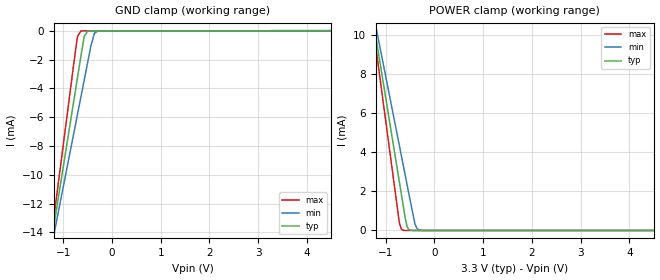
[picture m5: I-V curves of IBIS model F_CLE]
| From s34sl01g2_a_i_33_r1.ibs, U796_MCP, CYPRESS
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|   Model   F_CLE
[Model]   F_CLE
Model_type Input
Vinl =   0.6600V
Vinh =   2.6400V
   C_comp   1.3066pF   1.2854pF   1.3186pF
[Temperature Range]   25.0000   0.1050k   -40.0000
[Pullup Reference]   3.3000V   3.0000V   3.6000V
[Pulldown Reference]   0.0V   0.0V   0.0V
[POWER Clamp Reference]   3.3000V   3.0000V   3.6000V
[GND Clamp Reference]   0.0V   0.0V   0.0V
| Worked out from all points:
|   GND clamp passes 1 mA (typ) near -0.60 V on its own axis
|   POWER clamp passes 1 mA (typ) near -0.62 V on its own axis
[GND_clamp]
|Voltage   I(typ)   I(min)   I(max)
-3.3V     -58.25mA   -50.51mA   -68.01mA
-1.27V    -15.17mA   -15.49mA   -14.97mA
-1.2V     -13.69mA   -14.29mA   -13.14mA
-1.13V    -12.2mA    -13.08mA   -11.31mA
-710mV    -3.287mA   -5.833mA   -406.4uA
-640mV    -1.801mA   -4.625mA   -13.92uA
-570mV    -392.3uA   -3.417mA   -432.3nA
-500mV    -27.95uA   -2.21mA    -14.31nA
-430mV    -1.849uA   -1.002mA   -500.6pA
-360mV    -123.6nA   -162.7uA   -58.79pA
-290mV    -8.752nA   -19.51uA   -43.43pA
6.6V      39.73pA    16.96uA    36.6pA
[POWER_clamp]
|Voltage   I(typ)   I(min)   I(max)
-3.28V    41.85mA    36.71mA    48.13mA
-1.28V    11.09mA    11.42mA    10.82mA
-1.24V    10.47mA    10.92mA    10.07mA
-1.2V     9.856mA    10.41mA    9.323mA
-1.16V    9.241mA    9.904mA    8.577mA
-720mV    2.474mA    4.34mA     378.9uA
-680mV    1.859mA    3.834mA    63.12uA
-640mV    1.244mA    3.328mA    8.921uA
-560mV    171.5uA    2.316mA    167.4nA
-400mV    368.6nA    323.9uA    110.7pA
-280mV    3.503nA    9.212uA    50.14pA
6.6V      39.73pA    2.996nA    43.2pA
